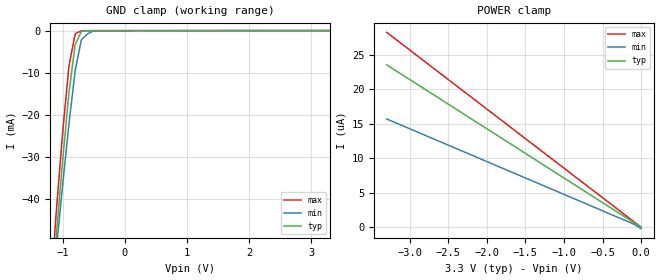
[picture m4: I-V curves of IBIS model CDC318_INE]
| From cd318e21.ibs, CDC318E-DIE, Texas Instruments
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|   Model CDC318_INE
[Model]   CDC318_INE
Model_type   Input
Polarity   Non-Inverting
Vinl = 0.8V
Vinh = 2.0V
Vmeas = 1.5V
| variable   typ   min   max
C_comp   3.2p   NA   NA
[Voltage range]   3.3   3.135   3.465
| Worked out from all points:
|   GND clamp passes 1 mA (typ) near -0.73 V on its own axis
[GND_Clamp]
|  Voltage   I(typ)   I(min)   I(max)
-3.3V     -477.4mA   -422.8mA   -533mA
-1.2V     -66.57mA   -66.77mA   -62.44mA
-1.1V     -48.31mA   -51.64mA   -42.57mA
-1V       -30.8mA    -36.62mA   -24.14mA
-900mV    -14.88mA   -22.3mA    -8.558mA
-800mV    -3.355mA   -9.579mA   -749uA
-700mV    -200.7uA   -2.192mA   -50.4uA
-600mV    -32.08uA   -782.8uA   -35.07uA
-500mV    -26.19uA   -20.75uA   -33.95uA
3.3V      -49.05nA   784.9nA    -1.413uA
[POWER_clamp]
|  Voltage   I(typ)   I(min)   I(max)
-3.3V     23.55uA    15.7uA     28.26uA
-2.8V     19.98uA    13.32uA    23.97uA
-100mV    713.5nA    475.7nA    856.3nA
0V        7.098pA    -216.4nA   7.32pA
